(* Low speed task. IEC 60870-5-101 unbalanced mode communication sample (controlled station) *)
PROGRAM P_MAIN_LowSpeed
VAR
	fbServer	: FB_IEC870_5_101S :=	( 	protPara := ( linkAddr 		:= 220,(* Link address *)
														eLinkAddrSize 	:= eIEC870_LinkAddr_OneOctet,(* Link address octet size *)
														eLinkMode 		:= eIEC870_LinkMode_Unbalanced(* Set unbalanced mode *) ), 
											sysPara := ( 	asduAddr 	:= 7,(* Common ASDU address *)
															nOrg 		:= 0,(* Originator address *)
															bCoro		:= TRUE,(* Enable/disable local counter freeze/reset command *)
															eCoroMode 	:= eIEC870_CoroMode_A,(* Counter interrogation mode *)
															bCoroReset	:= FALSE,(* Enable/disable local reset of counter values *)
															tCoro		:= T#60S,(* Local freeze and reset cycle time (Mode A and Mode B only) *)										
															bCyclic		:= TRUE,(* Enable/disable cyclic data *)
															tCyclic		:= T#60S,(* Cycle time of cyclic data *)														
															bDbgLink 	:= FALSE,(* Enable/disable serial link layer debug messages *) 
															bDbgAppl 	:= TRUE,(* Enable/disable application debug messages *) 
															eDbgAsdu 	:= eIEC870_FIFO_DBG_OFF,(* Enable/disable ASDU debug messages *) 
															asduFmt 	:= ( 	eCOTSize 		:= eIEC870_COT_OneOctet, 
																				eAsduAddrSize 	:= eIEC870_AsduAddr_OneOctet, 
																				eObjAddrSize 	:= eIEC870_ObjAddr_TwoOctets ) 
														) 
										);

	stProcData 		: ST_IEC870_5_101SProcData;(* Process data send to or received from IEC 60870-5-101 master device *)
	fbLog			: FB_IEC870_DebugLogFifo;(* Simple log buffer. We store/log here all our received slave data and other messages *)
	
	bSimulate 		: BOOL := FALSE;(* TRUE => Enable simulation of monitored data *)
	fbSimulate		: TON := ( IN := FALSE, PT := T#60S );
END_VAR

(* Execute slave instance *)
fbServer( hSerial := P_SerialComm_HighSpeed.hSerial, stProcData := stProcData, fbLog := fbLog );

(* Simulate monitoring data change *)
fbSimulate( IN := bSimulate );
IF fbSimulate.Q THEN
	fbSimulate( IN := FALSE );
	fbSimulate( IN := bSimulate );
	
	stProcData.stSiq100.SPI := NOT stProcData.stSiq100.SPI;
	stProcData.stSiq100.IV	:= NOT stProcData.stSiq100.IV;
 
	stProcData.stSiq101.SPI := NOT stProcData.stSiq101.SPI;
	stProcData.stSiq101.IV	:= NOT stProcData.stSiq101.IV;

	stProcData.stSiq102.SPI := NOT stProcData.stSiq102.SPI;
	stProcData.stSiq102.IV	:= NOT stProcData.stSiq102.IV;
	
	stProcData.stDiq200.DPI0 := NOT stProcData.stDiq200.DPI0;
	stProcData.stDiq200.DPI1 := NOT stProcData.stDiq200.DPI0;
	stProcData.stDiq200.IV	:= NOT stProcData.stDiq200.IV;
	
	stProcData.nVti300 		:= stProcData.nVti300 + 1;
	stProcData.stQds300.IV 	:= NOT stProcData.stQds300.IV;
	
	stProcData.nBsi400 		:= stProcData.nBsi400 + 1;
	stProcData.stQds400.IV 	:= NOT stProcData.stQds400.IV;
	
	stProcData.nNva500		:= stProcData.nNva500 + 1;
	stProcData.stQds500.IV	:= NOT stProcData.stQds500.IV;

	stProcData.nSva600		:= stProcData.nSva600 + 1;
	stProcData.stQds600.IV	:= NOT stProcData.stQds600.IV;

	stProcData.fSingle700	:= stProcData.fSingle700 + 1;
	stProcData.stQds700.IV	:= NOT stProcData.stQds700.IV;
	
	stProcData.nBcr800		:= stProcData.nBcr800 + 1;
	stProcData.stQcr800.IV	:= NOT stProcData.stQcr800.IV;

	stProcData.nBcr801		:= stProcData.nBcr801 + 1;
	stProcData.stQcr801.IV	:= NOT stProcData.stQcr801.IV;

	stProcData.nBcr802		:= stProcData.nBcr802 + 1;
	stProcData.stQcr802.IV	:= NOT stProcData.stQcr802.IV;
END_IF

END_PROGRAM
